{attribute 'call_after_init'}
FUNCTION_BLOCK FB_DS_IED_LD1_LLN0_DS5 EXTENDS FB_AcsiCommonDataSetClass
VAR
END_VAR

METHOD OnInit : BOOL
VAR
END_VAR
IF NOT DeleteAllMembers() THEN RETURN; END_IF
IF NOT AddMember(ipData:=fbIED.IEDLD1.MMXU1.TotW.mag, eFc:=E_AcsiFc.MX) THEN RETURN; END_IF
OnInit:= TRUE;
END_METHOD

END_FUNCTION_BLOCK
